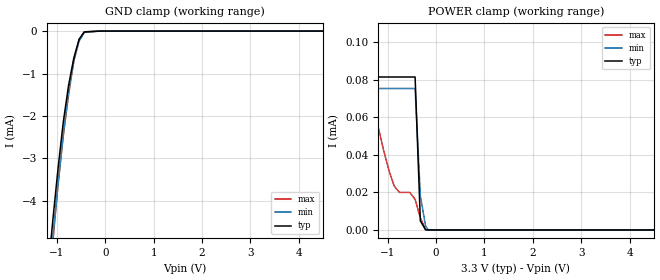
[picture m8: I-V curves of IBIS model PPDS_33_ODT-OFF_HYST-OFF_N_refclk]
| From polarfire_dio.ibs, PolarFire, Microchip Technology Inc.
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|   Model PPDS_33_ODT-OFF_HYST-OFF_N_refclk
[Model]   PPDS_33_ODT-OFF_HYST-OFF_N_refclk
Model_type   Input
Vinl =   0.675
Vinh =   0.925
|   typ   min   max
C_comp   2.671e-12   2.671e-12   2.761e-12
[Temperature Range]  25C   100C   -40C
[Voltage Range]  3.3   3.135   3.465
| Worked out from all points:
|   GND clamp passes 1 mA (typ) near -0.71 V on its own axis
[GND Clamp]
| Voltage   I(typ)   I(min)   I(max)
-3.3V     -52.75mA   -49.47mA   -59.64mA
-1.191V   -5.758mA   -6.191mA   -6.408mA
-1.083V   -4.447mA   -4.872mA   -4.952mA
-974.5mV  -3.225mA   -3.606mA   -3.588mA
-866.2mV  -2.135mA   -2.429mA   -2.451mA
-758mV    -1.279mA   -1.419mA   -1.499mA
-649.7mV  -634uA     -693.7uA   -709uA
-541.4mV  -197.9uA   -239.4uA   -196.4uA
-433.1mV  -18.64uA   -31.03uA   -18.18uA
-108.3mV  -1.607nA   -2.598nA   -6.538nA
6.6V      0A         0A         0A
[POWER Clamp]
| Voltage   I(typ)   I(min)   I(max)
-3.3V     277.2uA    202.6uA    360.3uA
-2.057V   132.9uA    104.3uA    176.6uA
-1.841V   106.7uA    83.54uA    143.5uA
-1.732V   94.14uA    76.98uA    127.4uA
-1.624V   81.93uA    75.39uA    111.5uA
-1.516V   81.53uA    75.39uA    96.13uA
-1.083V   81.53uA    75.39uA    42.31uA
-866.2mV  81.53uA    75.39uA    23.47uA
-433.1mV  81.53uA    75.39uA    16.32uA
-324.8mV  4.861uA    18.31uA    6.48uA
-216.6mV  92.15nA    2.076uA    79.05nA
6.6V      0A         0A         0A
